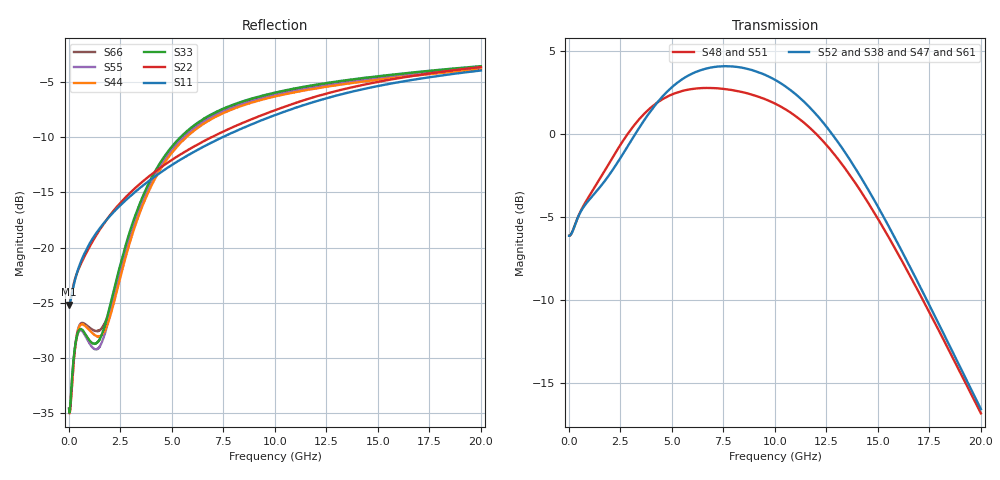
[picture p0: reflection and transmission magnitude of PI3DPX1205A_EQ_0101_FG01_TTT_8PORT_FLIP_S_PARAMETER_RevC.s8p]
! NPort=8 DATA=2000 NOISE=0 GROUPDELAY=0 COMPLEX_DATAFORMAT=POLAR
! NumOfBlock=1 NumOfParam=0
! .MODEL Smodel S TSTONEFILE=PI3DPX1205A_EQ_0101_FG01_TTT_8PORT_FLIP_S_PARAMETER_RevC.s8p TYPE=S
!  -- The above .MODEL line can be used for the S element in the netlist.
! The s parameter is extracted from the linear redriver, it is not bi-directional;
! only s(5,1)s(6,2)s(3,7)s(4,8) should be the insertion loss
!  Port definition:
!  Port1 = AIP
!  Port2 = AIN
!  Port3 = BOP
!  Port4 = BON
!  Port5 = AOP
!  Port6 = AON
!  Port7 = BIP
!  Port8 = BIN
# Hz S MA R  50
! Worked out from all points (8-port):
!   2000 points, 10 MHz to 20 GHz, reference 50 ohm
!   strongest paths, dB at 10 MHz, 5.01 GHz, 10.01 GHz, 15.01 GHz, 20 GHz:
!     S52: -6.1, 2.8, 3.3, -4.4, -16.6
!     S38: -6.1, 2.8, 3.2, -4.4, -16.6
!     S47: -6.1, 2.8, 3.3, -4.4, -16.5
!     S61: -6.1, 2.8, 3.3, -4.4, -16.5
!     S48: -6.1, 2.4, 1.8, -5.1, -16.9
!     S51: -6.1, 2.4, 1.8, -5.2, -16.9
!   lowest |S11| = -25.2 dB at 10 MHz (marker M1), VSWR 1.12, Z = 44.8 - j0.115 ohm
!   |S11| at or under -10 dB: start of sweep to 7.466 GHz
